(* Logix 5000 AddOnInstructionDefinition export HI6500_Faceplate_AOI; software revision 28.00; part 2 of 2 *)
(* tags used below, declared in another part *)
   Inp_hi6500 : _0102:Hardy6500Series_19FEEB66:I:0;
   Out_hi6500 : _0102:Hardy6500Series_74A2D67F:O:0;
   pm_4081 : DINT;
   pm_4082 : REAL;
   pm_4181 : REAL;
   pm_4182 : REAL;
   pm_2886 : REAL;
   pm_6182 : REAL;
   pm_6183 : REAL;
   pm_6301 : DINT;
   pm_6302 : REAL;
   pm_6381 : REAL;
   pm_6281 : DINT;
   pm_6282 : REAL;
   pm_6283 : REAL;
   wr_cell_sens : DINT;
   wr_zr_tol : DINT;
   wr_tr_off : DINT;
   wr_tr_amt : DINT;
   wr_cal_lo_wt : DINT;
   wr_span_wt : DINT;
   wr_az_enable : DINT;
   wr_az_tol : DINT;
   wr_warm_time : DINT;
   wr_iz_enable : DINT;
   wr_plusiz_tol : DINT;
   wr_minusiz_tol : DINT;
   save_op2_pm : INT;
   save_az_pm : INT;
   save_iz_pm : INT;
   save_tradcal_pm : INT;
   wr_cal_m_tol_2 : INT;
   wr_nvm_cmd : DINT;
   cmd_no : DINT;
   start_timer12 : BOOL;
   delay12 : TIMER;
   start_timer13 : BOOL;
   delay13 : TIMER;
   start_timer14 : BOOL;
   delay14 : TIMER;
   start_timer15 : BOOL;
   delay15 : TIMER;
   start_timer16 : BOOL;
   delay16 : TIMER;
   start_timer17 : BOOL;
   delay17 : TIMER;
   start_timer20 : BOOL;
   delay20 : TIMER;
   start_timer21 : BOOL;
   delay21 : TIMER;
   start_timer22 : BOOL;
   delay22 : TIMER;
   start_timer24 : BOOL;
   delay24 : TIMER;
   start_timer29 : BOOL;
   delay29 : TIMER;
   start_timer30 : BOOL;
   delay30 : TIMER;
   start_timer32 : BOOL;
   delay32 : TIMER;
   temp17 : BOOL;
   temp18 : BOOL;
   temp19 : BOOL;
   temp20 : BOOL;
   temp21 : BOOL;
   temp22 : BOOL;
   temp23 : BOOL;
   temp24 : BOOL;
   temp25 : BOOL;
   temp26 : BOOL;
   temp27 : BOOL;
   temp28 : BOOL;
   temp29 : BOOL;
(* HI6500_Faceplate_AOI, continued *)

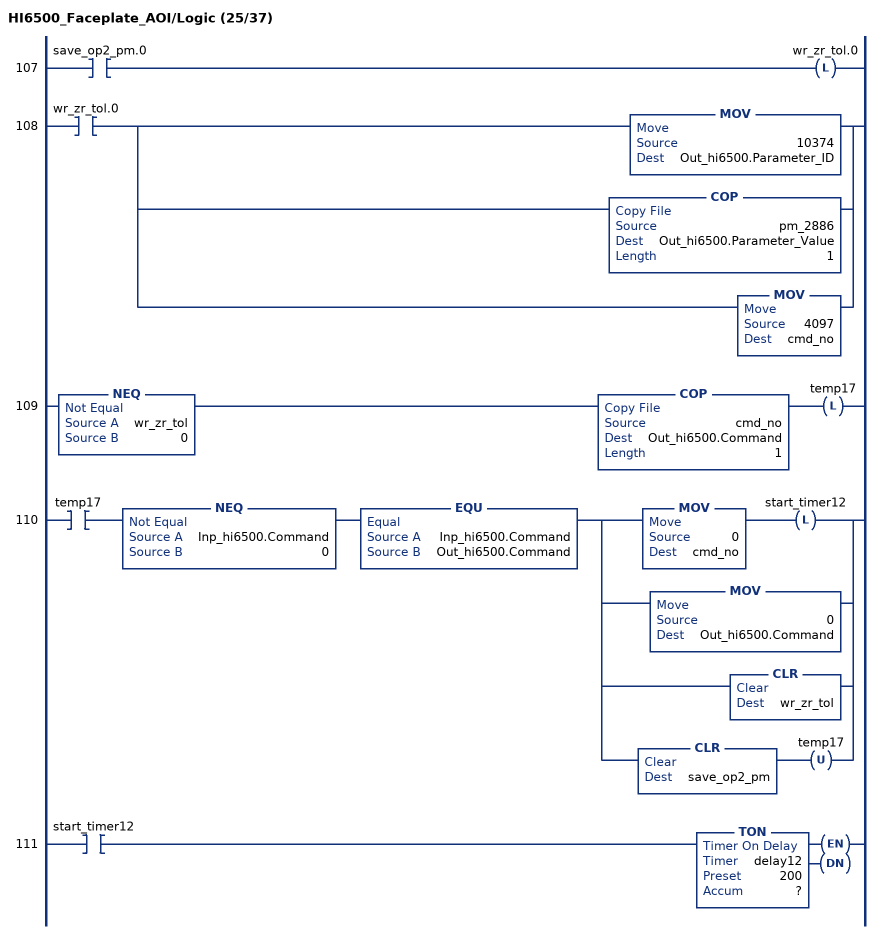
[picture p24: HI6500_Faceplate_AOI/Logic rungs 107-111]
   107: XIC(save_op2_pm.0)OTL(wr_zr_tol.0);
   108: XIC(wr_zr_tol.0)[MOV(10374,Out_hi6500.Parameter_ID) ,COP(pm_2886,Out_hi6500.Parameter_Value,1) ,MOV(4097,cmd_no) ];
   109: NEQ(wr_zr_tol,0)COP(cmd_no,Out_hi6500.Command,1)OTL(temp17);
   110: XIC(temp17)NEQ(Inp_hi6500.Command,0)EQU(Inp_hi6500.Command,Out_hi6500.Command)[MOV(0,cmd_no) OTL(start_timer12) ,MOV(0,Out_hi6500.Command) ,CLR(wr_zr_tol) ,CLR(save_op2_pm) OTU(temp17) ];
   111: XIC(start_timer12)TON(delay12,?,?);
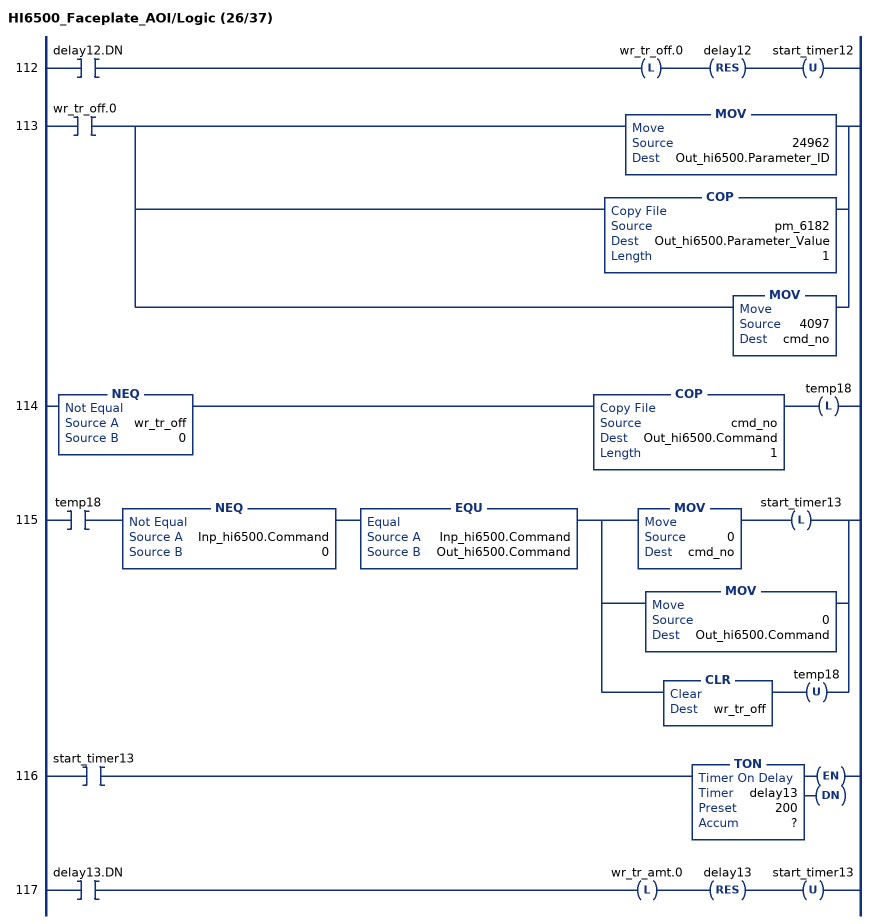
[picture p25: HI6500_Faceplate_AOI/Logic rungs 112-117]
   112: XIC(delay12.DN)OTL(wr_tr_off.0)RES(delay12)OTU(start_timer12);
   113: XIC(wr_tr_off.0)[MOV(24962,Out_hi6500.Parameter_ID) ,COP(pm_6182,Out_hi6500.Parameter_Value,1) ,MOV(4097,cmd_no) ];
   114: NEQ(wr_tr_off,0)COP(cmd_no,Out_hi6500.Command,1)OTL(temp18);
   115: XIC(temp18)NEQ(Inp_hi6500.Command,0)EQU(Inp_hi6500.Command,Out_hi6500.Command)[MOV(0,cmd_no) OTL(start_timer13) ,MOV(0,Out_hi6500.Command) ,CLR(wr_tr_off) OTU(temp18) ];
   116: XIC(start_timer13)TON(delay13,?,?);
   117: XIC(delay13.DN)OTL(wr_tr_amt.0)RES(delay13)OTU(start_timer13);
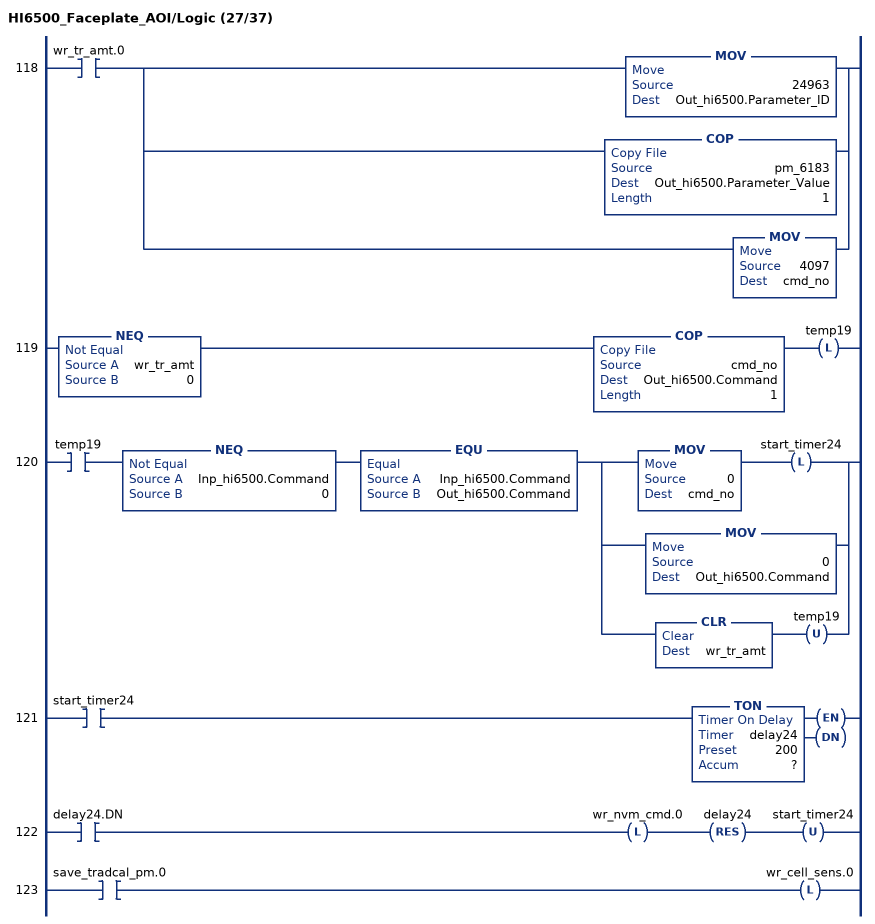
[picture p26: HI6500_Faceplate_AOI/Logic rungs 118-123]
   118: XIC(wr_tr_amt.0)[MOV(24963,Out_hi6500.Parameter_ID) ,COP(pm_6183,Out_hi6500.Parameter_Value,1) ,MOV(4097,cmd_no) ];
   119: NEQ(wr_tr_amt,0)COP(cmd_no,Out_hi6500.Command,1)OTL(temp19);
   120: XIC(temp19)NEQ(Inp_hi6500.Command,0)EQU(Inp_hi6500.Command,Out_hi6500.Command)[MOV(0,cmd_no) OTL(start_timer24) ,MOV(0,Out_hi6500.Command) ,CLR(wr_tr_amt) OTU(temp19) ];
   121: XIC(start_timer24)TON(delay24,?,?);
   122: XIC(delay24.DN)OTL(wr_nvm_cmd.0)RES(delay24)OTU(start_timer24);
   123: XIC(save_tradcal_pm.0)OTL(wr_cell_sens.0);
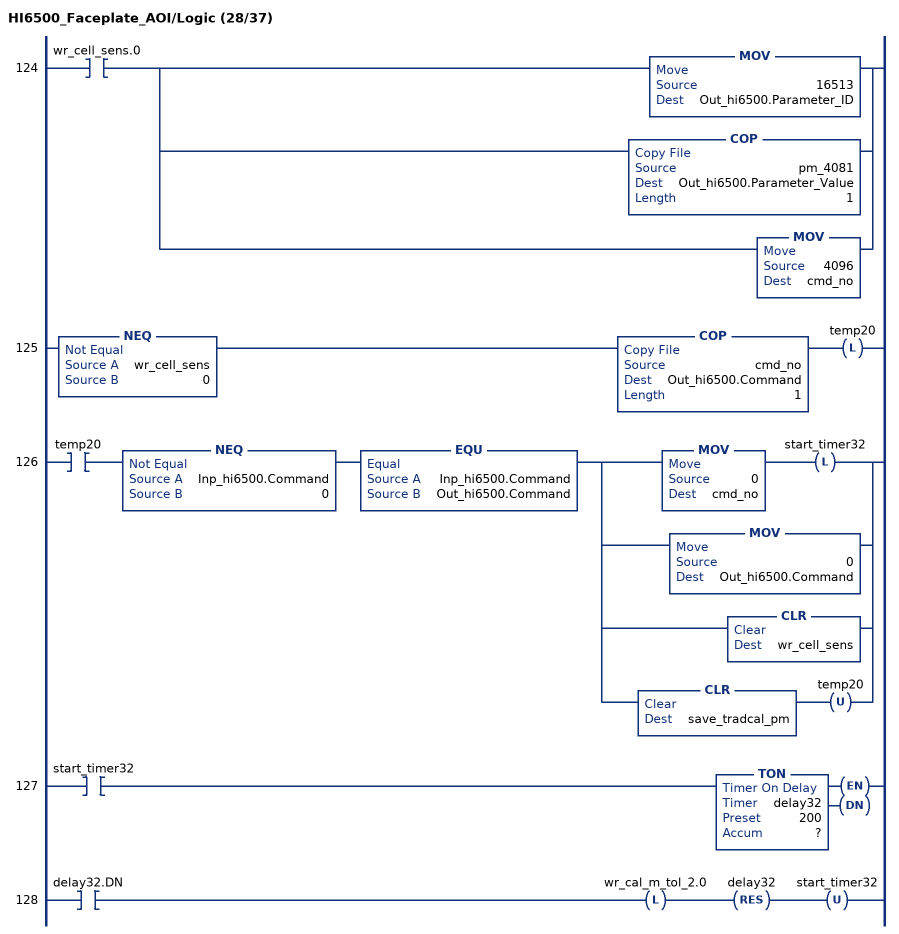
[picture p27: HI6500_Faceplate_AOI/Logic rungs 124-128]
   124: XIC(wr_cell_sens.0)[MOV(16513,Out_hi6500.Parameter_ID) ,COP(pm_4081,Out_hi6500.Parameter_Value,1) ,MOV(4096,cmd_no) ];
   125: NEQ(wr_cell_sens,0)COP(cmd_no,Out_hi6500.Command,1)OTL(temp20);
   126: XIC(temp20)NEQ(Inp_hi6500.Command,0)EQU(Inp_hi6500.Command,Out_hi6500.Command)[MOV(0,cmd_no) OTL(start_timer32) ,MOV(0,Out_hi6500.Command) ,CLR(wr_cell_sens) ,CLR(save_tradcal_pm) OTU(temp20) ];
   127: XIC(start_timer32)TON(delay32,?,?);
   128: XIC(delay32.DN)OTL(wr_cal_m_tol_2.0)RES(delay32)OTU(start_timer32);
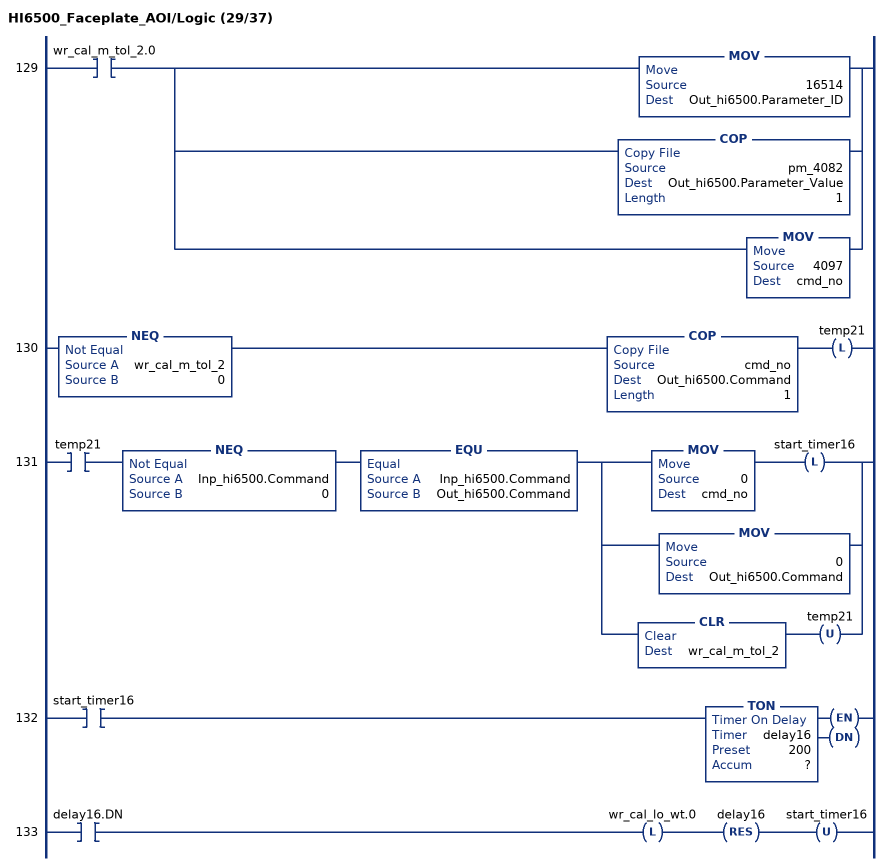
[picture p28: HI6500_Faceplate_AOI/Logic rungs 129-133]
   129: XIC(wr_cal_m_tol_2.0)[MOV(16514,Out_hi6500.Parameter_ID) ,COP(pm_4082,Out_hi6500.Parameter_Value,1) ,MOV(4097,cmd_no) ];
   130: NEQ(wr_cal_m_tol_2,0)COP(cmd_no,Out_hi6500.Command,1)OTL(temp21);
   131: XIC(temp21)NEQ(Inp_hi6500.Command,0)EQU(Inp_hi6500.Command,Out_hi6500.Command)[MOV(0,cmd_no) OTL(start_timer16) ,MOV(0,Out_hi6500.Command) ,CLR(wr_cal_m_tol_2) OTU(temp21) ];
   132: XIC(start_timer16)TON(delay16,?,?);
   133: XIC(delay16.DN)OTL(wr_cal_lo_wt.0)RES(delay16)OTU(start_timer16);
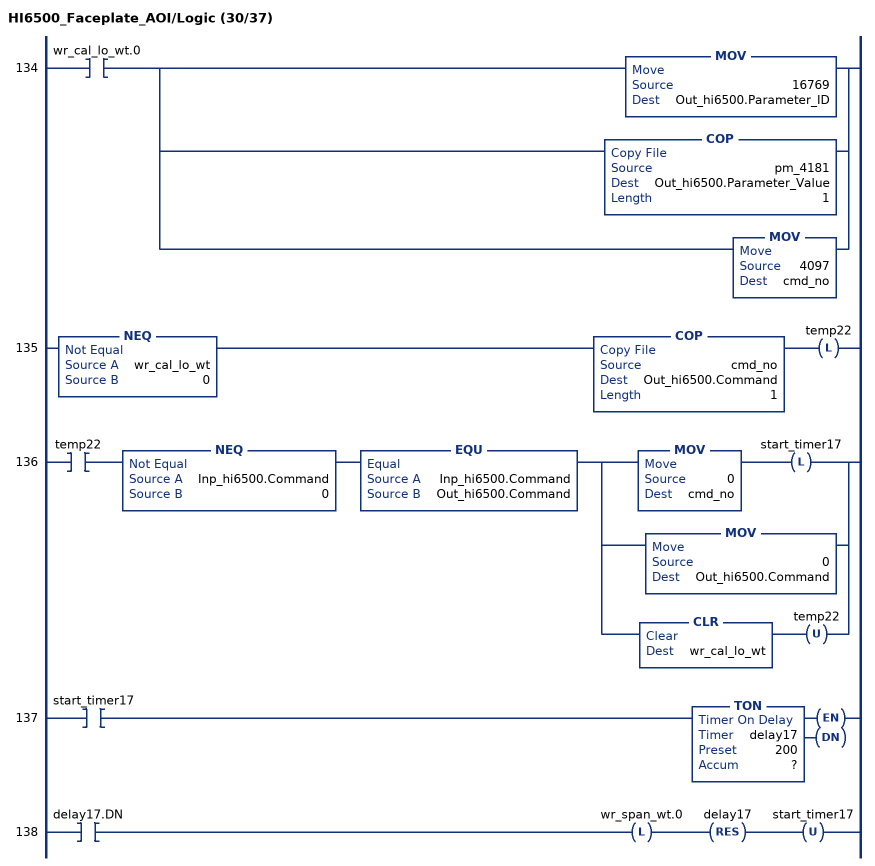
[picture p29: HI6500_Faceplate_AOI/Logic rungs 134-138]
   134: XIC(wr_cal_lo_wt.0)[MOV(16769,Out_hi6500.Parameter_ID) ,COP(pm_4181,Out_hi6500.Parameter_Value,1) ,MOV(4097,cmd_no) ];
   135: NEQ(wr_cal_lo_wt,0)COP(cmd_no,Out_hi6500.Command,1)OTL(temp22);
   136: XIC(temp22)NEQ(Inp_hi6500.Command,0)EQU(Inp_hi6500.Command,Out_hi6500.Command)[MOV(0,cmd_no) OTL(start_timer17) ,MOV(0,Out_hi6500.Command) ,CLR(wr_cal_lo_wt) OTU(temp22) ];
   137: XIC(start_timer17)TON(delay17,?,?);
   138: XIC(delay17.DN)OTL(wr_span_wt.0)RES(delay17)OTU(start_timer17);
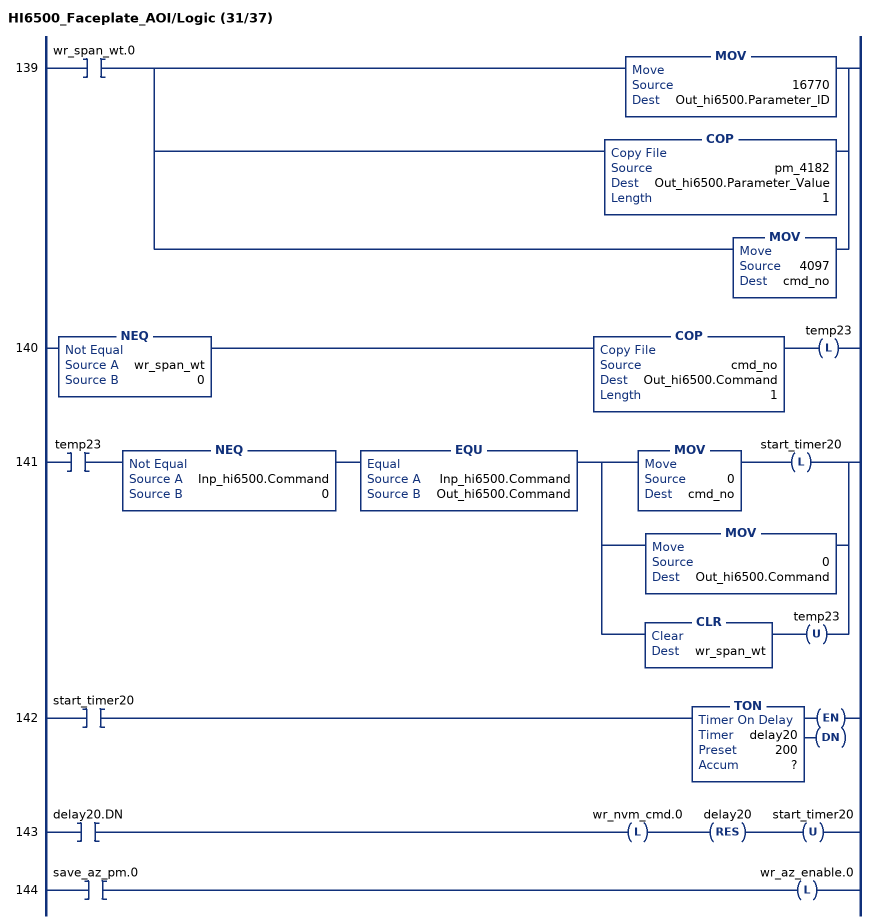
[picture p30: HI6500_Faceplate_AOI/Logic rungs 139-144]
   139: XIC(wr_span_wt.0)[MOV(16770,Out_hi6500.Parameter_ID) ,COP(pm_4182,Out_hi6500.Parameter_Value,1) ,MOV(4097,cmd_no) ];
   140: NEQ(wr_span_wt,0)COP(cmd_no,Out_hi6500.Command,1)OTL(temp23);
   141: XIC(temp23)NEQ(Inp_hi6500.Command,0)EQU(Inp_hi6500.Command,Out_hi6500.Command)[MOV(0,cmd_no) OTL(start_timer20) ,MOV(0,Out_hi6500.Command) ,CLR(wr_span_wt) OTU(temp23) ];
   142: XIC(start_timer20)TON(delay20,?,?);
   143: XIC(delay20.DN)OTL(wr_nvm_cmd.0)RES(delay20)OTU(start_timer20);
   144: XIC(save_az_pm.0)OTL(wr_az_enable.0);
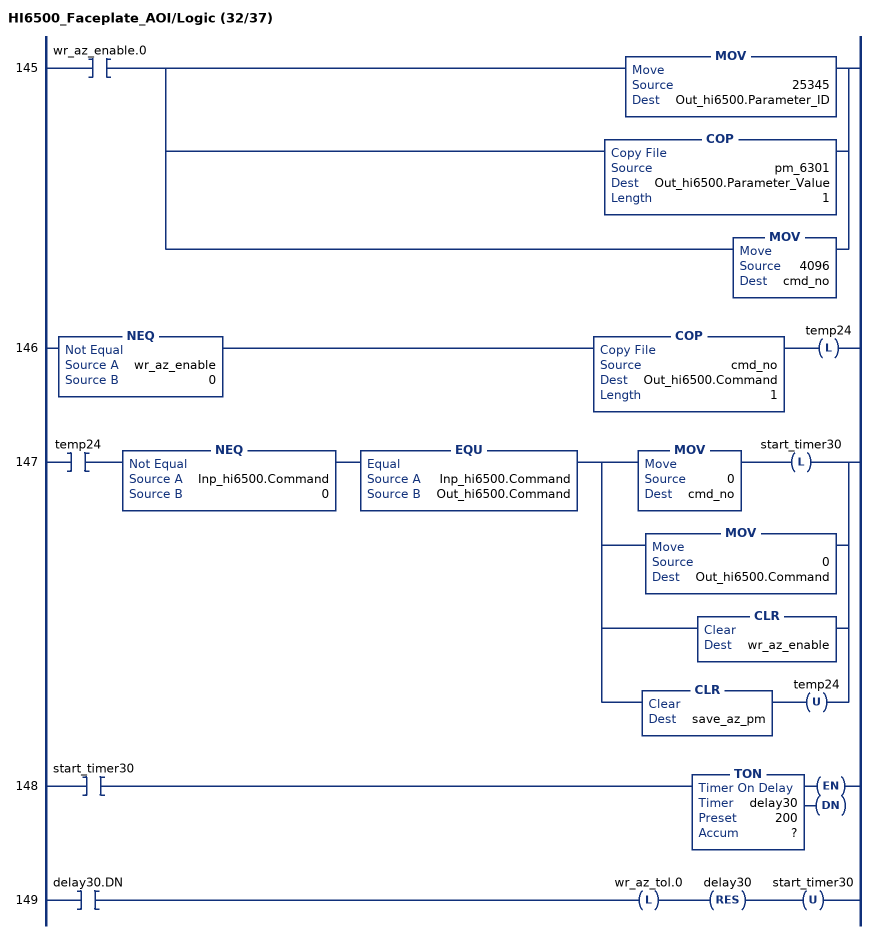
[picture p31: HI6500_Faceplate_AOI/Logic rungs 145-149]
   145: XIC(wr_az_enable.0)[MOV(25345,Out_hi6500.Parameter_ID) ,COP(pm_6301,Out_hi6500.Parameter_Value,1) ,MOV(4096,cmd_no) ];
   146: NEQ(wr_az_enable,0)COP(cmd_no,Out_hi6500.Command,1)OTL(temp24);
   147: XIC(temp24)NEQ(Inp_hi6500.Command,0)EQU(Inp_hi6500.Command,Out_hi6500.Command)[MOV(0,cmd_no) OTL(start_timer30) ,MOV(0,Out_hi6500.Command) ,CLR(wr_az_enable) ,CLR(save_az_pm) OTU(temp24) ];
   148: XIC(start_timer30)TON(delay30,?,?);
   149: XIC(delay30.DN)OTL(wr_az_tol.0)RES(delay30)OTU(start_timer30);
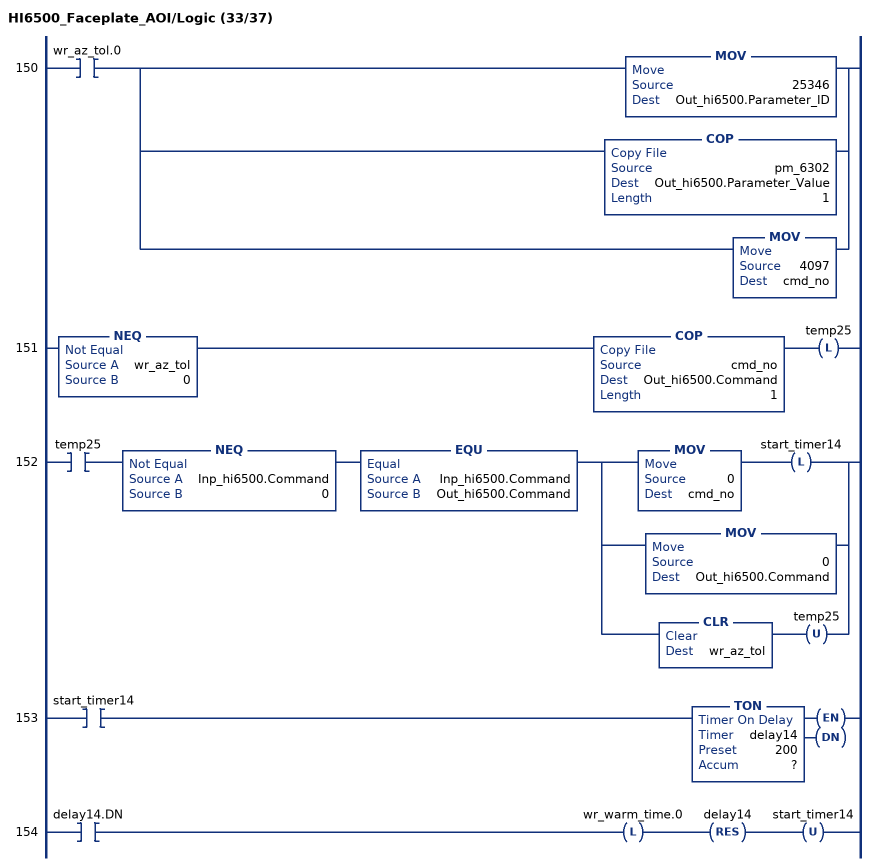
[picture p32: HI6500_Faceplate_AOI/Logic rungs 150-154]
   150: XIC(wr_az_tol.0)[MOV(25346,Out_hi6500.Parameter_ID) ,COP(pm_6302,Out_hi6500.Parameter_Value,1) ,MOV(4097,cmd_no) ];
   151: NEQ(wr_az_tol,0)COP(cmd_no,Out_hi6500.Command,1)OTL(temp25);
   152: XIC(temp25)NEQ(Inp_hi6500.Command,0)EQU(Inp_hi6500.Command,Out_hi6500.Command)[MOV(0,cmd_no) OTL(start_timer14) ,MOV(0,Out_hi6500.Command) ,CLR(wr_az_tol) OTU(temp25) ];
   153: XIC(start_timer14)TON(delay14,?,?);
   154: XIC(delay14.DN)OTL(wr_warm_time.0)RES(delay14)OTU(start_timer14);
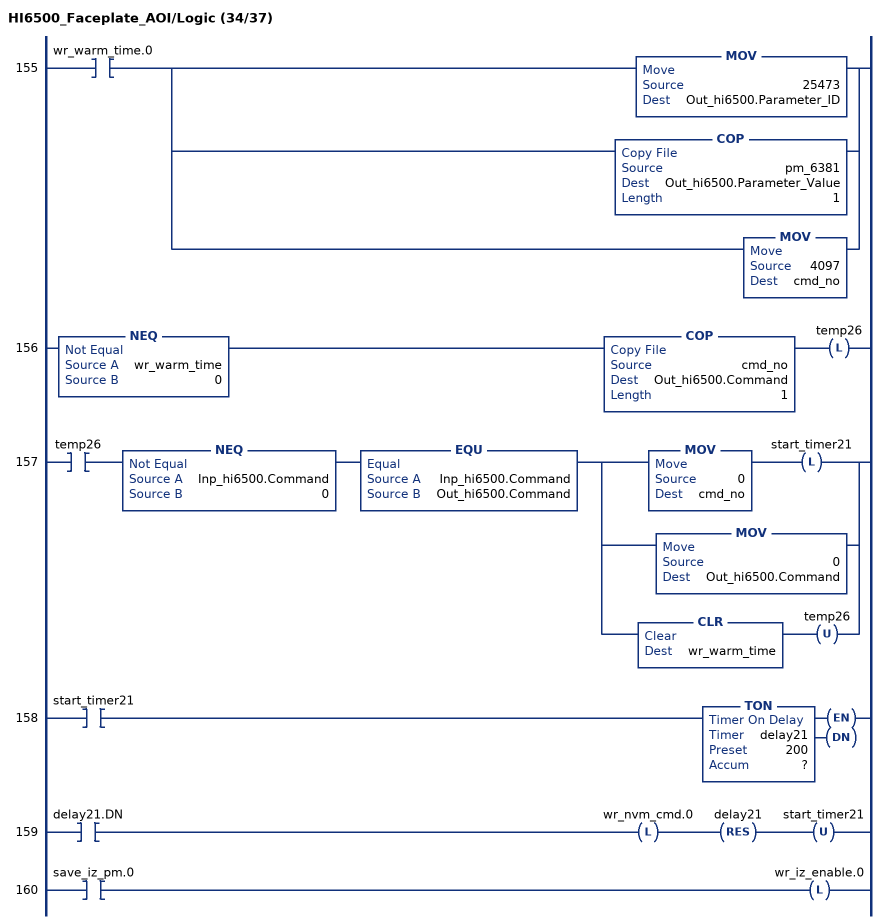
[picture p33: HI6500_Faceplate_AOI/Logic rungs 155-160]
   155: XIC(wr_warm_time.0)[MOV(25473,Out_hi6500.Parameter_ID) ,COP(pm_6381,Out_hi6500.Parameter_Value,1) ,MOV(4097,cmd_no) ];
   156: NEQ(wr_warm_time,0)COP(cmd_no,Out_hi6500.Command,1)OTL(temp26);
   157: XIC(temp26)NEQ(Inp_hi6500.Command,0)EQU(Inp_hi6500.Command,Out_hi6500.Command)[MOV(0,cmd_no) OTL(start_timer21) ,MOV(0,Out_hi6500.Command) ,CLR(wr_warm_time) OTU(temp26) ];
   158: XIC(start_timer21)TON(delay21,?,?);
   159: XIC(delay21.DN)OTL(wr_nvm_cmd.0)RES(delay21)OTU(start_timer21);
   160: XIC(save_iz_pm.0)OTL(wr_iz_enable.0);
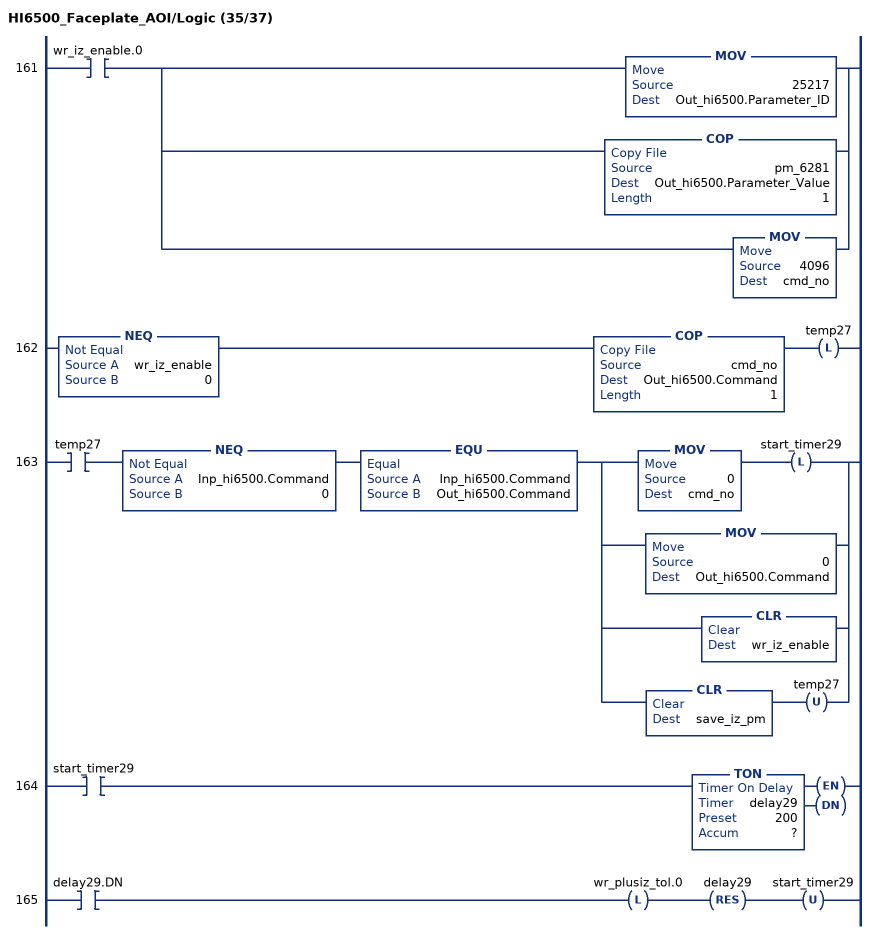
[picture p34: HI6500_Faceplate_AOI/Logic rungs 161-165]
   161: XIC(wr_iz_enable.0)[MOV(25217,Out_hi6500.Parameter_ID) ,COP(pm_6281,Out_hi6500.Parameter_Value,1) ,MOV(4096,cmd_no) ];
   162: NEQ(wr_iz_enable,0)COP(cmd_no,Out_hi6500.Command,1)OTL(temp27);
   163: XIC(temp27)NEQ(Inp_hi6500.Command,0)EQU(Inp_hi6500.Command,Out_hi6500.Command)[MOV(0,cmd_no) OTL(start_timer29) ,MOV(0,Out_hi6500.Command) ,CLR(wr_iz_enable) ,CLR(save_iz_pm) OTU(temp27) ];
   164: XIC(start_timer29)TON(delay29,?,?);
   165: XIC(delay29.DN)OTL(wr_plusiz_tol.0)RES(delay29)OTU(start_timer29);
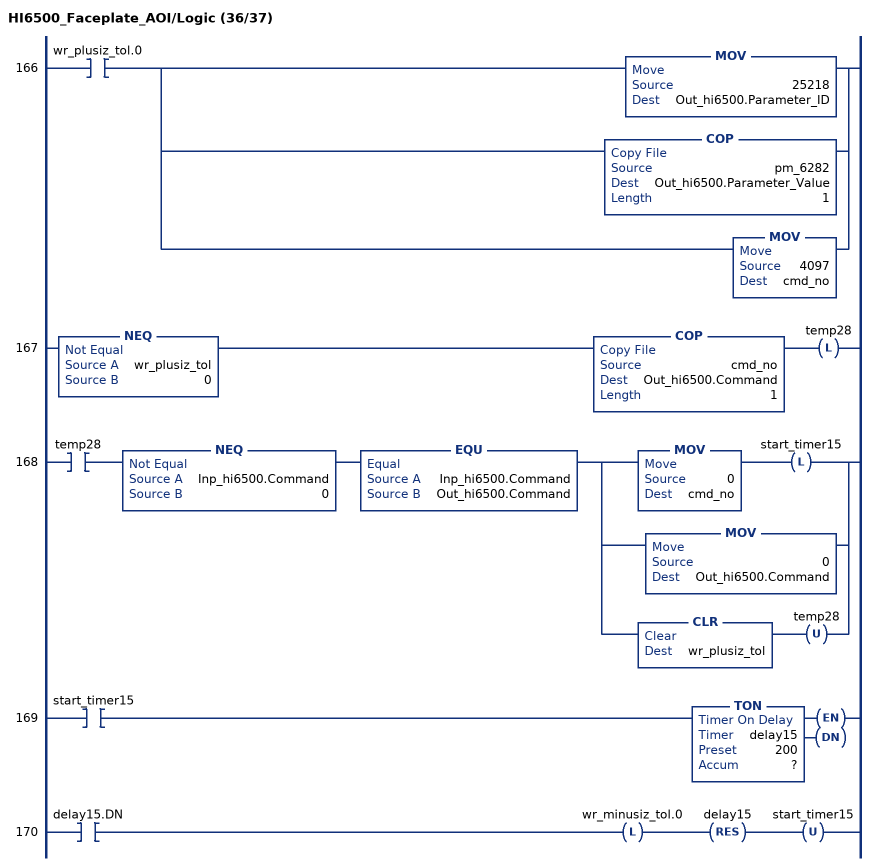
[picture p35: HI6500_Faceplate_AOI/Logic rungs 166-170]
   166: XIC(wr_plusiz_tol.0)[MOV(25218,Out_hi6500.Parameter_ID) ,COP(pm_6282,Out_hi6500.Parameter_Value,1) ,MOV(4097,cmd_no) ];
   167: NEQ(wr_plusiz_tol,0)COP(cmd_no,Out_hi6500.Command,1)OTL(temp28);
   168: XIC(temp28)NEQ(Inp_hi6500.Command,0)EQU(Inp_hi6500.Command,Out_hi6500.Command)[MOV(0,cmd_no) OTL(start_timer15) ,MOV(0,Out_hi6500.Command) ,CLR(wr_plusiz_tol) OTU(temp28) ];
   169: XIC(start_timer15)TON(delay15,?,?);
   170: XIC(delay15.DN)OTL(wr_minusiz_tol.0)RES(delay15)OTU(start_timer15);
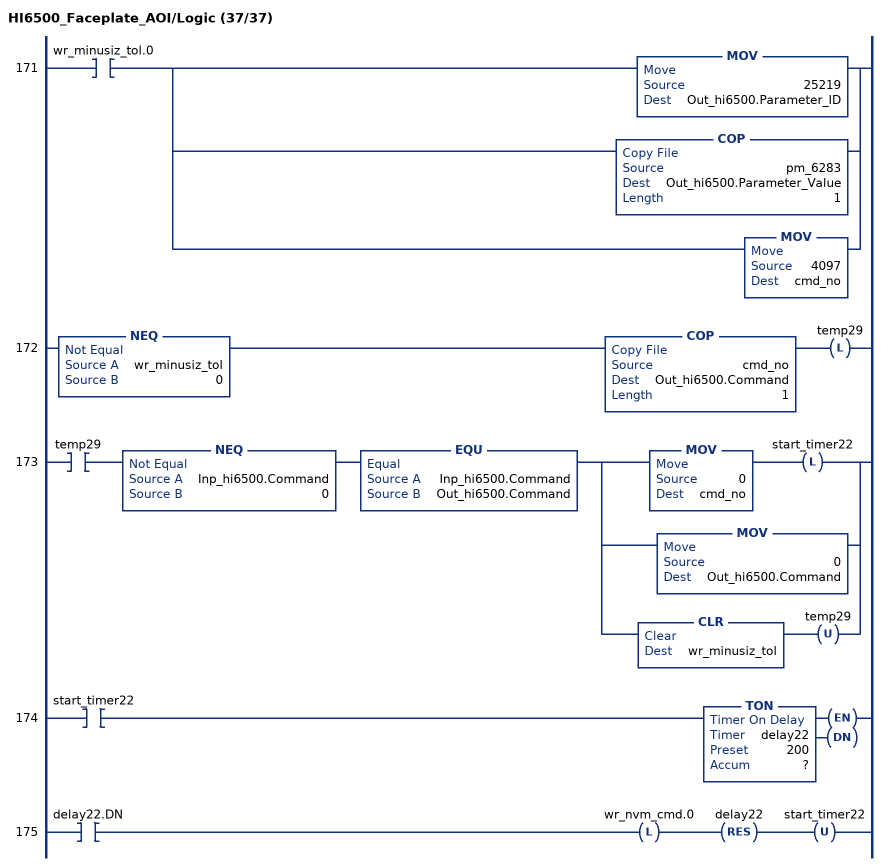
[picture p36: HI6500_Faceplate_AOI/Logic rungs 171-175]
   171: XIC(wr_minusiz_tol.0)[MOV(25219,Out_hi6500.Parameter_ID) ,COP(pm_6283,Out_hi6500.Parameter_Value,1) ,MOV(4097,cmd_no) ];
   172: NEQ(wr_minusiz_tol,0)COP(cmd_no,Out_hi6500.Command,1)OTL(temp29);
   173: XIC(temp29)NEQ(Inp_hi6500.Command,0)EQU(Inp_hi6500.Command,Out_hi6500.Command)[MOV(0,cmd_no) OTL(start_timer22) ,MOV(0,Out_hi6500.Command) ,CLR(wr_minusiz_tol) OTU(temp29) ];
   174: XIC(start_timer22)TON(delay22,?,?);
   175: XIC(delay22.DN)OTL(wr_nvm_cmd.0)RES(delay22)OTU(start_timer22);
END_ROUTINE
END_ADD_ON_INSTRUCTION
